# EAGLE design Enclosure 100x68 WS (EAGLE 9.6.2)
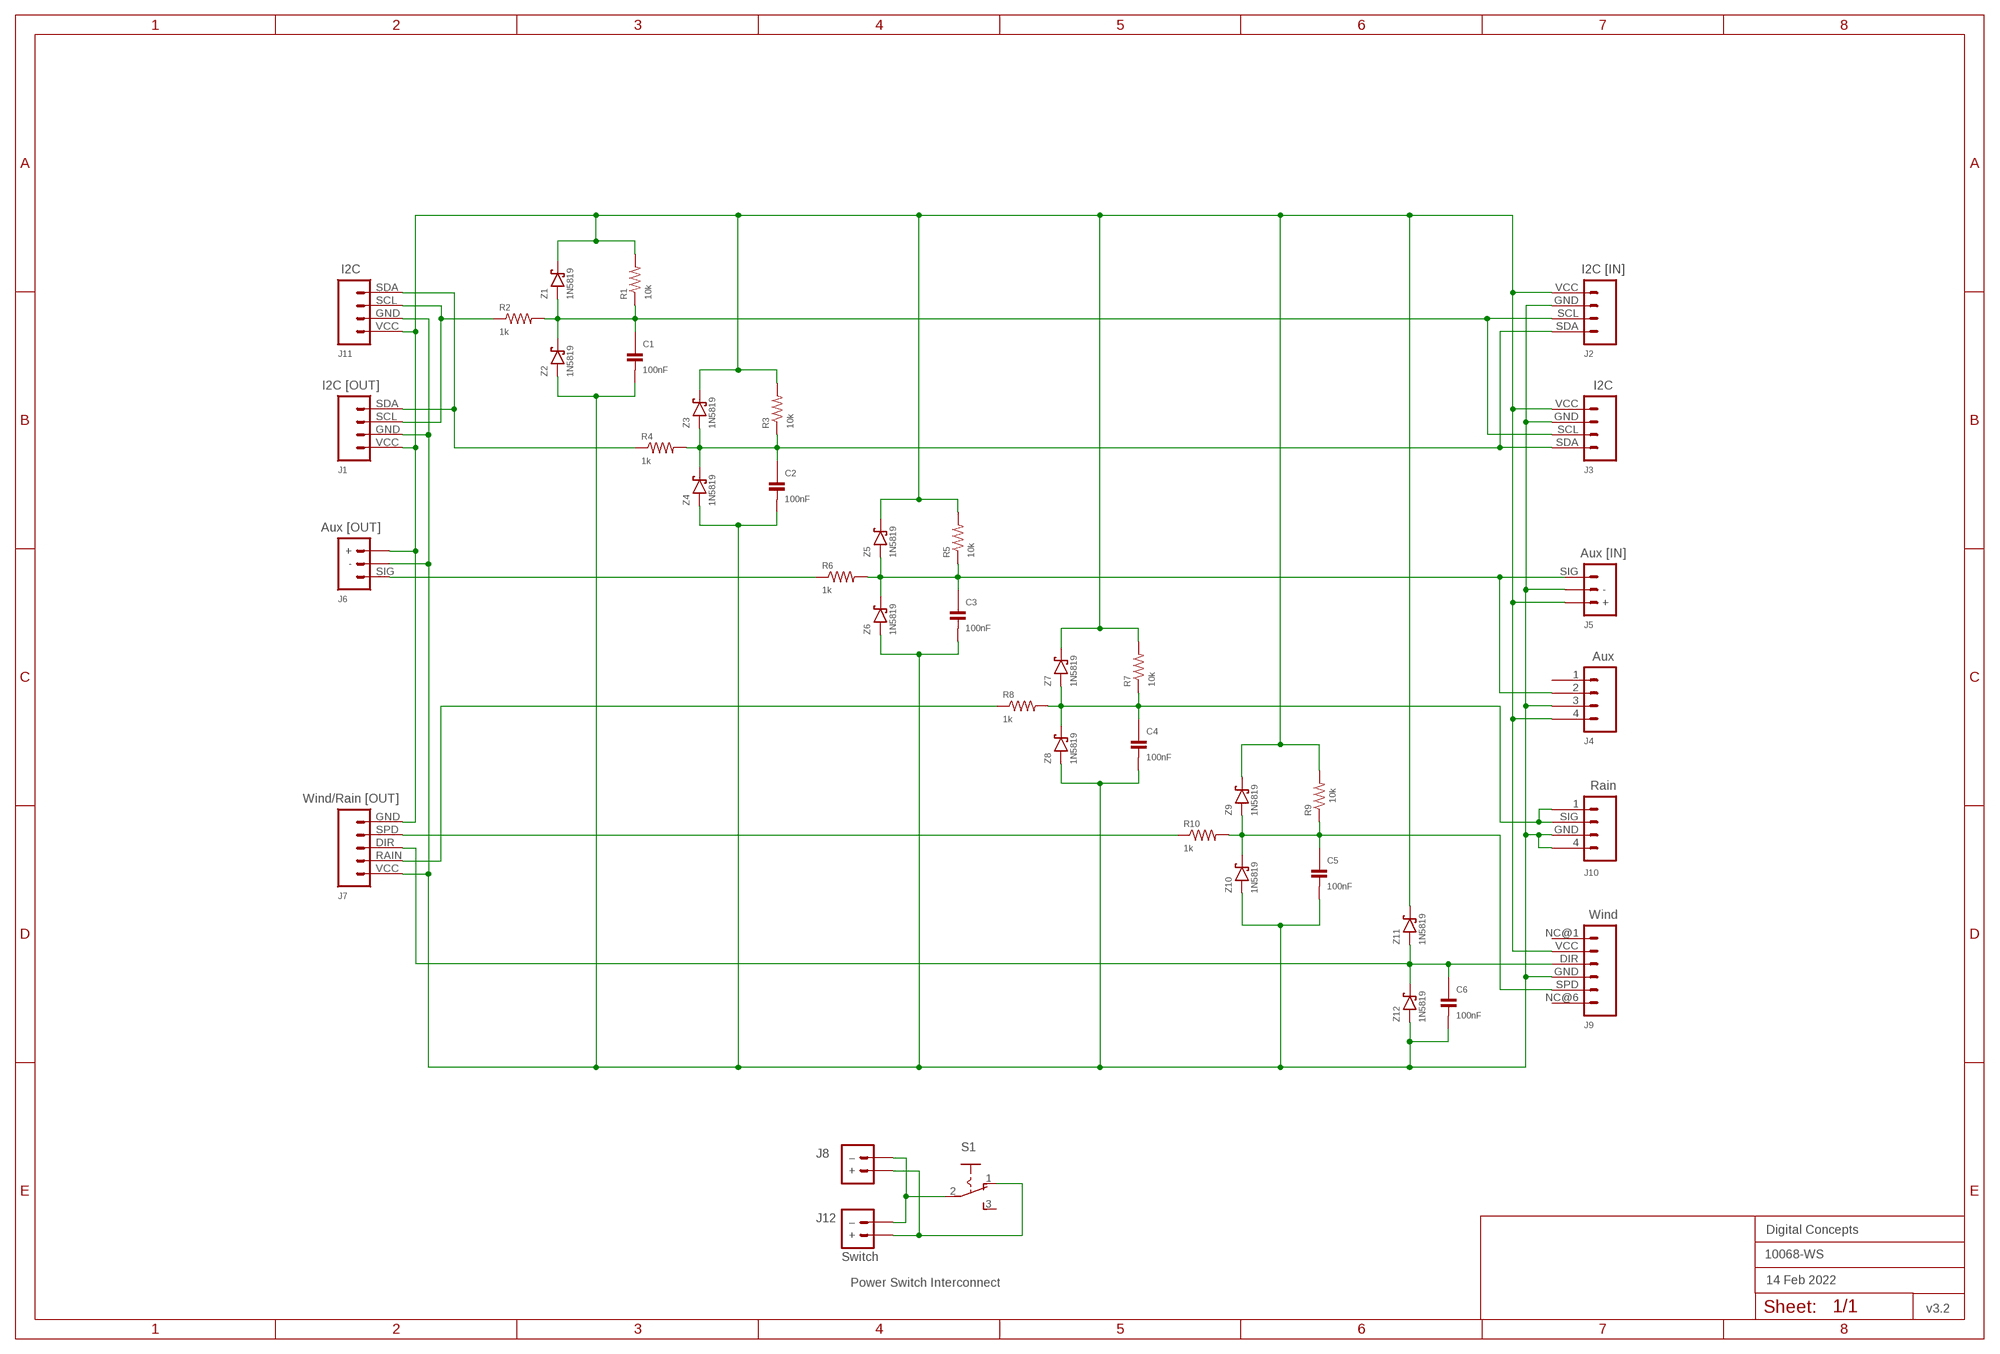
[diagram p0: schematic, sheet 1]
FRAME2 (A3L-LOC): DATE: 14 Feb 2022; OWNER: Digital Concepts; TITLE: 10068-WS; VERSION: v3.2

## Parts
C1  100nF  CAPACITOR-0805  [C0805]
C2  100nF  CAPACITOR-0805  [C0805]
C3  100nF  CAPACITOR-0805  [C0805]
C4  100nF  CAPACITOR-0805  [C0805]
C5  100nF  CAPACITOR-0805  [C0805]
C6  100nF  CAPACITOR-0805  [C0805]
J1  I2C [OUT]  JST-PH2.0-4-DUAL-I2C  [JST-PH2.0-4-DUAL-I2C]
J2  I2C [IN]  JST-PH2.0-4-VERTICAL-I2C  [JST-PH2.0-4-VERTICAL-I2C]
J3  I2C  RJ11-6P4C-VERTICAL-I2C  [RJ11-4-VERTICAL-I2C]
J4  Aux  RJ11-6P4C-VERTICAL  [RJ11-4-VERTICAL]
J5  Aux [IN]  JST-PH2.0-3-VERTICAL-SIG  [JST-PH2.0-3-VERTICAL-SIG]
J6  Aux [OUT]  JST-PH2.0-3-DUAL-SIG  [JST-PH2.0-3-DUAL-SIG]
J7  Wind/Rain [OUT]  JST-PH2.0-5-DUAL-WEATHER  [JST-PH2.0-5-DUAL-WEATHER]
J8  Switch  JST-PH2.0-2-VERTICAL-POWER  [JST-PH2.0-2-VERTICAL=POWER]
J9  Wind  RJ11-6P6C-VERTICAL-WIND  [RJ11-6-VERTICAL-WIND]
J10  Rain  RJ11-6P4C-VERTICAL-RAIN  [RJ11-4-VERTICAL-RAIN]
J11  I2C  HEADER-1X4-I2C  [CONN_04-I2C]
J12  Switch  JST-PH2.0-2-HORIZONTAL-POWERJST-PTH-2  [JST-PH2.0-2-HORIZONTAL-POWER]
R1  10k  RESISTORR0805  [R0805]
R2  1k  RESISTORR0805  [R0805]
R3  10k  RESISTORR0805  [R0805]
R4  1k  RESISTORR0805  [R0805]
R5  10k  RESISTORR0805  [R0805]
R6  1k  RESISTORR0805  [R0805]
R7  10k  RESISTORR0805  [R0805]
R8  1k  RESISTORR0805  [R0805]
R9  10k  RESISTORR0805  [R0805]
R10  1k  RESISTORR0805  [R0805]
S1  SWITCH-SLIDE-SPDT  [SWITCH-SPDT-PTH]
Z1  1N5819  DIODE-SCHOTTKY-1N5819  [SOD-123]
Z2  1N5819  DIODE-SCHOTTKY-1N5819  [SOD-123]
Z3  1N5819  DIODE-SCHOTTKY-1N5819  [SOD-123]
Z4  1N5819  DIODE-SCHOTTKY-1N5819  [SOD-123]
Z5  1N5819  DIODE-SCHOTTKY-1N5819  [SOD-123]
Z6  1N5819  DIODE-SCHOTTKY-1N5819  [SOD-123]
Z7  1N5819  DIODE-SCHOTTKY-1N5819  [SOD-123]
Z8  1N5819  DIODE-SCHOTTKY-1N5819  [SOD-123]
Z9  1N5819  DIODE-SCHOTTKY-1N5819  [SOD-123]
Z10  1N5819  DIODE-SCHOTTKY-1N5819  [SOD-123]
Z11  1N5819  DIODE-SCHOTTKY-1N5819  [SOD-123]
Z12  1N5819  DIODE-SCHOTTKY-1N5819  [SOD-123]

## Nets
GND: C1.2 C2.2 C3.2 C4.2 C5.2 C6.2 J1.GND J2.GND J3.GND J4.3 J5.- J6.- J7.VCC J9.GND J10.4 J10.GND J11.GND Z2.A Z4.A Z6.A Z8.A Z10.A Z12.A
N$1: J7.RAIN R8.1
N$2: J1.SCL J11.SCL R2.1
N$3: J1.SDA J11.SDA R4.1
N$4: C6.1 J7.DIR J9.DIR Z11.A Z12.C
N$5: J7.SPD R10.1
N$7: C4.1 J10.1 J10.SIG R7.1 R8.2 Z7.A Z8.C
N$8: C2.1 J2.SDA J3.SDA R3.1 R4.2 Z3.A Z4.C
N$9: J6.SIG R6.1
N$11: C1.1 J2.SCL J3.SCL R1.1 R2.2 Z1.A Z2.C
N$14: J8.-(–) J12.-(–) S1.2(P)
N$15: C3.1 J4.2 J5.SIG R5.1 R6.2 Z5.A Z6.C
N$16: J8.+ J12.+ S1.1(O)
N$29: C5.1 J9.SPD R9.1 R10.2 Z9.A Z10.C
VCC: J1.VCC J2.VCC J3.VCC J4.4 J5.+ J6.+ J7.GND J9.VCC J11.VCC R1.2 R3.2 R5.2 R7.2 R9.2 Z1.C Z3.C Z5.C Z7.C Z9.C Z11.C
Unconnected: J4.1 J9.NC@1 J9.NC@6 S1.3(S)

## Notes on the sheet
- Power Switch Interconnect

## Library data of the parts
C1-C6 = digitalconcepts:CAPACITOR-0805: 0805 Capacitor
J1 = digitalconcepts:JST-PH2.0-4-DUAL-I2C: PH2.0 4P I2C Dual Connector
J2 = digitalconcepts:JST-PH2.0-4-VERTICAL-I2C: PH2.0 4P I2C Vertical Connector
J3 = digitalconcepts:RJ11-6P4C-VERTICAL-I2C: RJ11-6P4C-Vertical PCB Socket
J4 = digitalconcepts:RJ11-6P4C-VERTICAL: RJ11-6P4C-Vertical PCB Socket
J5 = digitalconcepts:JST-PH2.0-3-VERTICAL-SIG: PH2.0 3P Vertical Connector (Sig)
J6 = digitalconcepts:JST-PH2.0-3-DUAL-SIG: PH2.0 3P Dual Sig Horizontal on top, vertical on bottom
J7 = digitalconcepts:JST-PH2.0-5-DUAL-WEATHER: PH2.0 5P Dual Connector
J8 = digitalconcepts:JST-PH2.0-2-VERTICAL-POWER: JST PH2.0 2P PTH Connector (Power)
J9 = digitalconcepts:RJ11-6P6C-VERTICAL-WIND: RJ11-6P6C-Vertical PCB Socket
J10 = digitalconcepts:RJ11-6P4C-VERTICAL-RAIN: RJ11-6P4C-Vertical PCB Socket
J11 = digitalconcepts:HEADER-1X4-I2C: I2C Interface [Pin 1 Vcc] 4-Pin Header
J12 = digitalconcepts:JST-PH2.0-2-HORIZONTAL-POWER: PH2.0 2P Right Angle PCB Connector; PROD_ID: CONN-09863; SKU: PRT-09914
R1-R10 = digitalconcepts:RESISTOR: Resistor; SPICEPREFIX: R
S1 = digitalconcepts:SWITCH-SLIDE-SPDT: Mini Sliding Switch SPDT
Z1-Z12 = digitalconcepts:DIODE-SCHOTTKY-1N5819: 1N5819 Schottky Diode SOD-123

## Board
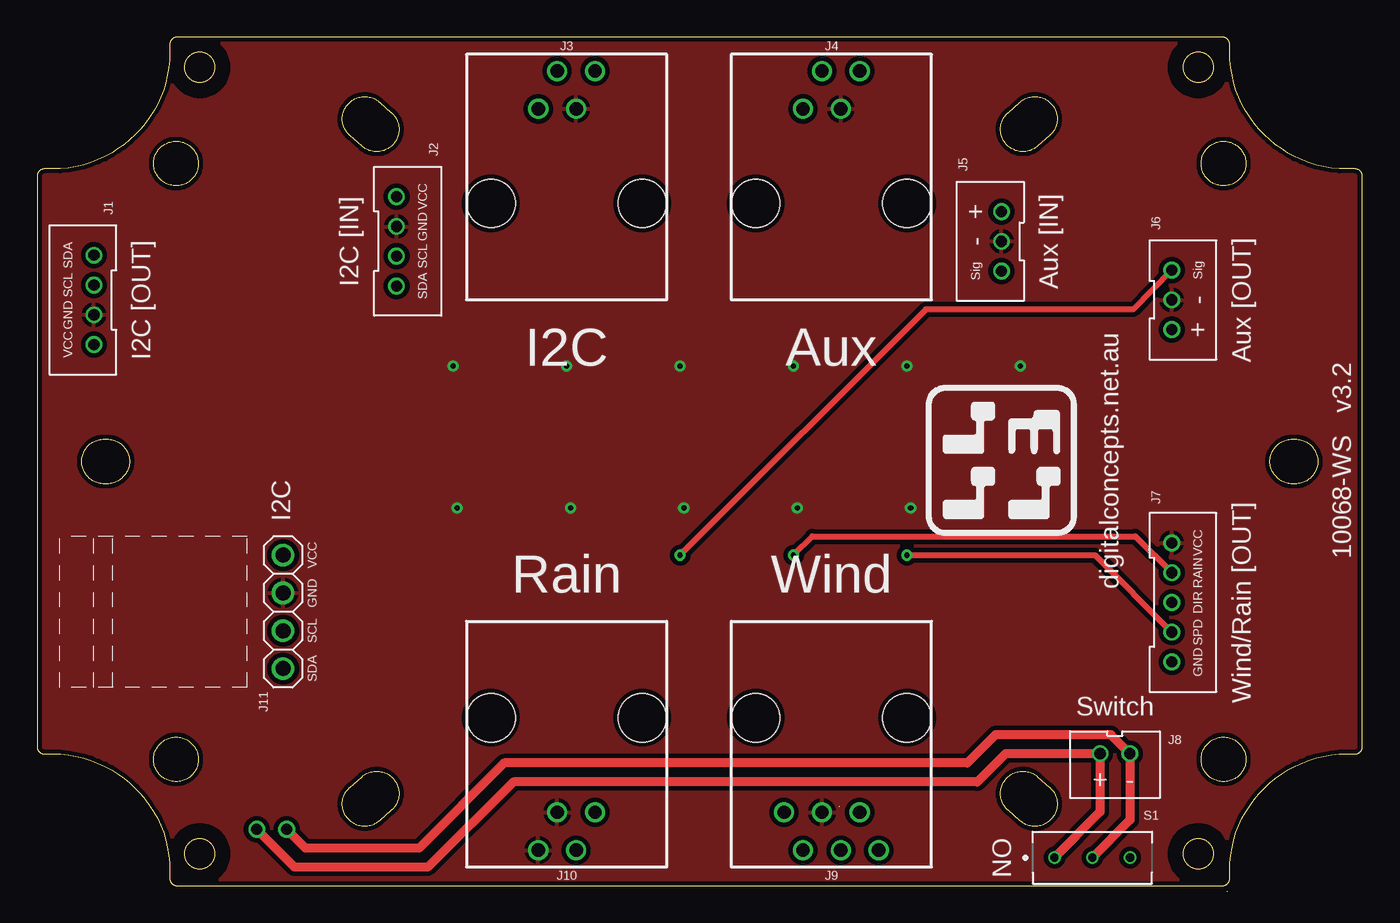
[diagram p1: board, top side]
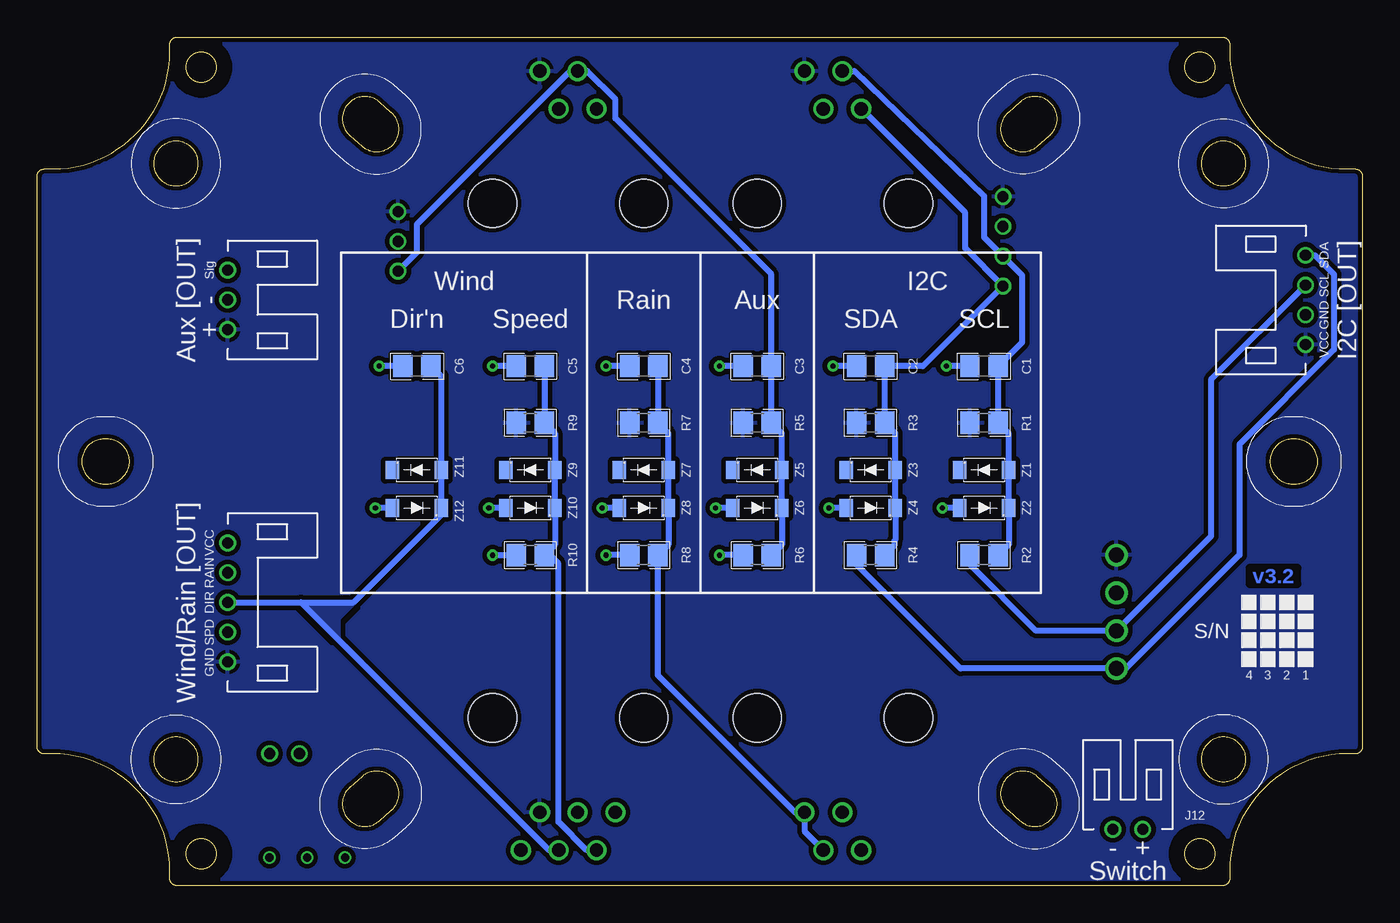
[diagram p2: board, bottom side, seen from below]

Size 89 x 57 mm. Coordinates in mm from the lower left corner, seen from the top.
Outline: 1238 segments
Outline: circle at 77.98,2.14 radius 1.02
Outline: circle at 10.92,2.14 radius 1.02
Outline: circle at 10.92,54.97 radius 1.02
Outline: circle at 77.98,54.97 radius 1.02
Copper layers (1*16): Top 0.035mm / dielectric 1.5mm / Bottom 0.035mm
Design rules "default *": minimum track width 6mil, minimum drill 0.35mm, track to track 6mil, track to pad 6mil, pad to pad 6mil, via to via 6mil, smd to smd 6mil, copper to edge 6mil, drill to drill 6mil, minimum pad ring 1mil, minimum via ring 8mil, stop-mask expansion 4mil, vias tented up to drill 0mil, thermal gap 10mil

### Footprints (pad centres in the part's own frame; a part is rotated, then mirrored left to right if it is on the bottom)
C0805 = smd 1.3 x 1.5: 1 -0.95,0; 2 0.95,0
JST-PH2.0-4-DUAL-I2C = drill 0.75: GND -1,0; SCL 1,0; SDA 3,0; VCC -3,0
JST-PH2.0-4-VERTICAL-I2C = drill 0.75: GND 1,0; SCL -1,0; SDA -3,0; VCC 3,0
RJ11-4-VERTICAL-I2C = drill 0.9: GND 0.635,4.58; SCL -0.635,7.12; SDA -1.905,4.58; VCC 1.905,7.12 | hole 3.25: -5.08,-1.77; 5.08,-1.77
RJ11-4-VERTICAL = drill 0.9: 1 -1.905,4.58; 2 -0.635,7.12; 3 0.635,4.58; 4 1.905,7.12 | hole 3.25: -5.08,-1.77; 5.08,-1.77
JST-PH2.0-3-VERTICAL-SIG = drill 0.75: + -2,0; - 0,0; SIG 2,0
JST-PH2.0-3-DUAL-SIG = drill 0.75: + 2,0; - 0,0; SIG -2,0
JST-PH2.0-5-DUAL-WEATHER = drill 0.75: DIR 0,0; GND 4,0; RAIN -2,0; SPD 2,0; VCC -4,0
JST-PH2.0-2-VERTICAL=POWER = drill 0.75: + -1,0; - 1,0
RJ11-6-VERTICAL-WIND = drill 0.9: DIR -0.635,7.12; GND 0.635,4.58; NC@1 -3.175,7.12; NC@6 3.175,4.58; SPD 1.905,7.12; VCC -1.905,4.58 | hole 3.25: -5.08,-1.77; 5.08,-1.77
RJ11-4-VERTICAL-RAIN = drill 0.9: 1 -1.905,4.58; 4 1.905,7.12; GND 0.635,4.58; SIG -0.635,7.12 | hole 3.25: -5.08,-1.77; 5.08,-1.77
CONN_04-I2C = drill 1 pad 1.524: GND 2.54,0; SCL 5.08,0; SDA 7.62,0; VCC 0,0
JST-PH2.0-2-HORIZONTAL-POWER = drill 0.75: + 1,0; - -1,0
R0805 = smd 1.3 x 1.5: 1 -0.95,0; 2 0.95,0
SWITCH-SPDT-PTH = drill 0.55: 1 -2.54,0; 2 0,0; 3 2.54,0
SOD-123 = smd 0.91 x 1.22: A -1.65,0; C 1.65,0

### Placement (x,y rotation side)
C1  25.4,34.91 180 bottom
C2  33.02,34.91 180 bottom
C3  40.64,34.91 180 bottom
C4  48.26,34.91 180 bottom
C5  55.88,34.91 180 bottom
C6  63.5,34.91 180 bottom
J1  3.81,39.35 90 bottom
J2  24.13,43.29 90 top
J3  35.56,47.61 0 top
J4  53.34,47.61 0 top
J5  64.77,43.29 270 top
J6  76.2,39.35 270 bottom
J7  76.2,19.03 270 bottom
J8  72.39,8.87 0 top
J9  53.34,9.51 180 top
J10  35.56,9.51 180 top
J11  16.51,22.21 270 top
J12  15.75,3.79 0 bottom
R1  25.4,31.1 180 bottom
R2  25.4,22.21 0 bottom
R3  33.02,31.1 180 bottom
R4  33.02,22.21 0 bottom
R5  40.64,31.1 180 bottom
R6  40.64,22.21 0 bottom
R7  48.26,31.1 180 bottom
R8  48.26,22.21 0 bottom
R9  55.88,31.1 180 bottom
R10  55.88,22.21 0 bottom
S1  70.87,1.89 0 top
Z1  25.4,27.92 180 bottom
Z2  25.4,25.38 0 bottom
Z3  33.02,27.92 180 bottom
Z4  33.02,25.38 0 bottom
Z5  40.64,27.92 180 bottom
Z6  40.64,25.38 0 bottom
Z7  48.26,27.92 180 bottom
Z8  48.26,25.38 0 bottom
Z9  55.88,27.92 180 bottom
Z10  55.88,25.38 0 bottom
Z11  63.5,27.92 180 bottom
Z12  63.5,25.38 0 bottom

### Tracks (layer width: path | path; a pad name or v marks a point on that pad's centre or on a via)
$X0
  cutout Bottom: 10.92,52.94 arc180 10.92,57 arc180
$X1
  cutout Bottom: 77.98,52.94 arc180 77.98,57 arc180
$X2
  cutout Bottom: 77.98,0.11 arc180 77.98,4.17 arc180
$X3
  cutout Bottom: 10.92,0.11 arc180 10.92,4.17 arc180
$X4
  cutout Top: 10.92,52.94 arc180 10.92,57 arc180
$X5
  cutout Top: 77.98,52.94 arc180 77.98,57 arc180
$X6
  cutout Top: 77.98,0.11 arc180 77.98,4.17 arc180
$X7
  cutout Top: 10.92,0.11 arc180 10.92,4.17 arc180
GND  (via drill 0.35)
  Bottom 0.406: C4.2 v50.8,34.91 | C3.2 v43.18,34.91 | C5.2 v58.42,34.91 | C6.2 v66.04,34.91 | C1.2 v27.94,34.91 | C2.2 v35.56,34.91 | Z2.A v28.19,25.38 | Z4.A v35.81,25.38 | Z6.A v43.43,25.38 | Z8.A v51.05,25.38 | Z10.A v58.67,25.38 | Z12.A v66.29,25.38
  pour Top (isolate 0.305, rank 2): 90.6,-1.82 90.6,58.97 -1.64,58.97 -1.64,-1.82
N$1  (via drill 0.35)
  Top 0.406: v50.8,22.21 52.07,23.48 73.76,23.48 J7.RAIN
  Bottom 0.406: R8.1 v50.8,22.21
N$2
  Bottom 0.406: J1.SCL 10.16,34 10.16,23.48 J11.SCL 21.91,17.13 26.35,21.57 R2.1
N$3
  Bottom 0.406: J1.SDA 3.18,42.35 1.91,41.08 1.91,36 8.26,29.65 8.26,22.21 15.88,14.59 J11.SDA 26.99,14.59 33.97,21.57 R4.1
N$4
  Bottom 0.406: J9.DIR 54.64,2.39 71.28,19.03 | C6.1 61.85,34.21 Z11.A Z12.C 61.85,24.93 67.75,19.03 71.28,19.03 | J7.DIR 71.28,19.03
  pour Bottom: 67.74,19.03 68.83,17.94 68.83,16.59 71.27,19.03
N$5  (via drill 0.35)
  Top 0.406: v58.42,22.21 71.03,22.21 J7.SPD
  Bottom 0.406: v58.42,22.21 R10.1
N$7
  Bottom 0.406: C4.1 R7.1 46.61,30.4 Z7.A Z8.C 46.61,22.91 R8.2 47.31,14.14 38.1,4.93 J10.1 37.47,3.66 J10.SIG
N$8
  Bottom 0.406: J3.SDA 26.67,45.2 26.67,42.83 J2.SDA 29.51,34.91 C2.1 R3.1 31.37,30.4 Z3.A Z4.C 31.37,23.22 31.44,23.16 31.44,22.84 R4.2
N$9  (via drill 0.35)
  Top 0.406: J6.SIG 73.62,38.72 59.69,38.72 v43.18,22.21
  Bottom 0.406: R6.1 v43.18,22.21
N$11
  Bottom 0.406: J3.SCL 34.11,54.73 25.4,46.34 25.4,43.56 J2.SCL 22.86,41.02 22.86,36.5 C1.1 R1.1 23.75,30.4 Z1.A Z2.C 23.75,22.91 R2.2
N$14
  Top 0.61: J12.- 18.02,2.52 25.64,2.52 31.35,8.24 62.47,8.24 64.37,10.14 72.12,10.14 J8.- 73.39,4.41 S1.2
N$15
  Bottom 0.406: R6.2 38.99,22.91 Z6.C Z5.A 38.99,30.4 R5.1 C3.1 39.69,41.08 50.17,51.55 50.17,52.82 52.07,54.73 J4.2 53.21,54.73 63.5,44.43 63.5,42.56 J5.SIG
N$16
  Top 0.61: J12.+ 17.29,1.25 26.22,1.25 31.99,6.97 63.14,6.97 65.04,8.87 J8.+ 71.39,4.95 S1.1
N$29
  Bottom 0.406: J9.SPD 52.1,2.39 53.99,4.28 53.99,21.65 54.93,22.59 R10.2 54.23,22.91 Z10.C Z9.A 54.23,30.4 R9.1 C5.1
VCC
  pour Bottom (isolate 0.305, rank 5): 89.6,-0.82 89.6,57.97 -0.64,57.97 -0.64,-0.82

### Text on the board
Bottom: v3.2
tPlace: digitalconcepts.net.au | 10068-WS v3.2
bPlace: S/N | 1 | 2 | 3 | 4
tNames: VCC | GND | SCL | SDA | Switch | ON
bNames: I2C | Wind | I2C [OUT] | Aux | Rain | Aux [OUT] | SCL | SDA | Speed | Dir'n | Wind/Rain [OUT]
